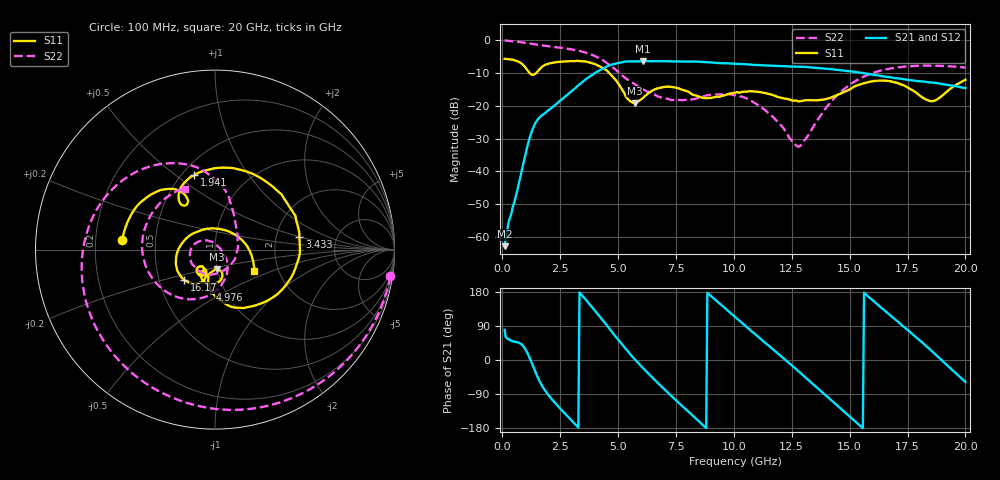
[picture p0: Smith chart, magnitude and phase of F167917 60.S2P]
!  2-Port S-parameters saved by WinCal
! VAR MeasName=S-Parameters (CALIBRATED_DATA) read from VNA (N5242A)
! VAR MeasDate=2016-11-22 9:02:58
! VAR NAME=F167917 60
! VAR FILENAME=F167917 60.S2P
! VAR DATE=2016-11-22 9:02:58
! VAR PHYS_PORTS=1,2
# Hz S DB R 50
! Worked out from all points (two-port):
!   401 points, 100 MHz to 20 GHz, reference 50 ohm
!   highest |S21| = -6.41 dB at 6.07 GHz (marker M1); lowest = -62.8 dB at 100 MHz (marker M2)
!   |S21| within 3 dB of the highest: 4.15 GHz to 14.87 GHz (10.72 GHz wide, 113 % of centre)
!   lowest |S11| = -19.1 dB at 5.722 GHz (marker M3), VSWR 1.25, Z = 49.9 - j11.1 ohm
!   |S11| at or under -10 dB: 1.175 GHz to 1.465 GHz (289.7 MHz wide, 21.9 % of centre); 4.617 GHz to end of sweep
!   |S22| runs from -32.6 to -0.1 dB; largest |S21 - S12| = 0.0033
!   S11 on the Smith chart (normalised r, x): 100 MHz: 0.32, +0.05; 1.941 GHz: 0.58, +0.58; 3.433 GHz: 2.72, +0.48; 4.976 GHz: 0.86, -0.41; 16.17 GHz: 0.67, -0.24; 20 GHz: 1.51, -0.37
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1e8  -5.71 174.2  -62.83 79.7  -62.26 80.4  -0.10 -8.7
9.4575e8  -7.85 123.6  -36.41 33.2  -36.41 33.3  -0.78 -73.9
1.3935e9  -10.45 125.3  -25.76 -25.6  -25.76 -25.4  -1.28 -103.2
1.94075e9  -7.34 105.7  -21.64 -88.4  -21.63 -88.4  -1.80 -134.1
2.687e9  -6.51 59.2  -17.37 -140.3  -17.38 -140.3  -2.49 -171.7
3.43325e9  -6.46 8.2  -12.92 171.1  -12.92 171.3  -3.47 152.1
4.22925e9  -8.10 -49.8  -9.12 112.9  -9.10 113.0  -5.67 112.8
4.9755e9  -12.88 -96.5  -7.03 55.8  -7.00 55.7  -9.46 80.4
5.72175e9  -19.15 -84.1  -6.47 1.7  -6.46 1.6  -13.50 59.4
6.07e9  -17.63 -73.2  -6.41 -20.8  -6.41 -20.8  -14.97 49.5
6.7665e9  -14.64 -87.2  -6.41 -63.4  -6.40 -63.4  -17.29 22.9
7.5625e9  -14.60 -110.9  -6.49 -109.7  -6.49 -109.7  -18.26 -22.6
8.50775e9  -17.25 -120.0  -6.58 -163.0  -6.54 -163.1  -17.55 -84.0
1.005e10  -16.02 -115.2  -7.20 113.7  -7.19 113.8  -16.84 -164.5
1.189075e10  -17.35 -133.9  -7.89 17.9  -7.85 17.9  -24.86 123.9
1.278625e10  -18.67 -127.2  -8.13 -29.2  -8.10 -29.2  -32.57 47.2
1.338325e10  -18.36 -121.0  -8.34 -61.9  -8.31 -61.8  -27.01 -17.4
1.49255e10  -15.30 -109.3  -9.45 -144.8  -9.40 -145.0  -13.99 -79.5
1.616925e10  -12.38 -135.7  -10.72 148.4  -10.71 148.4  -9.62 -125.1
1.67165e10  -12.50 -154.3  -11.27 120.1  -11.32 120.0  -8.70 -143.8
1.855725e10  -18.61 82.3  -12.90 23.3  -12.93 23.2  -7.81 159.2
2e10  -12.10 -28.0  -14.59 -57.9  -14.50 -57.5  -8.41 116.5
